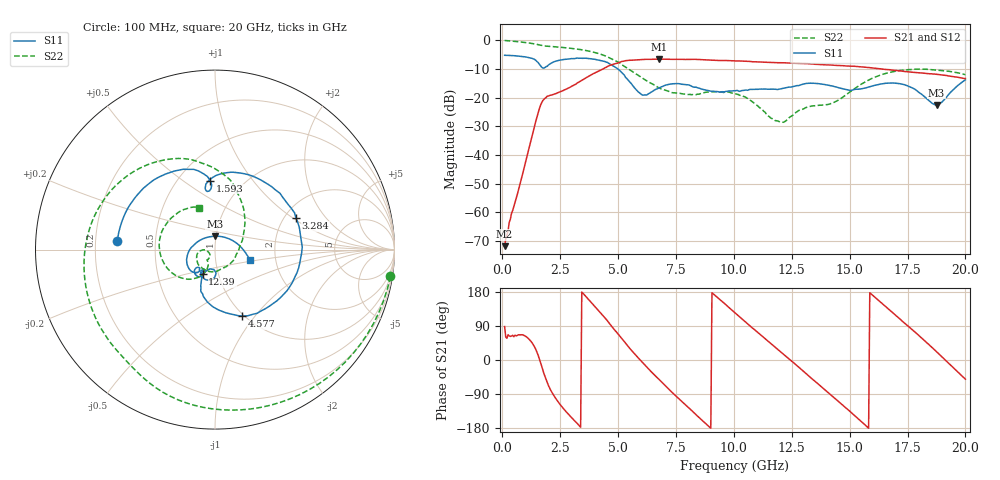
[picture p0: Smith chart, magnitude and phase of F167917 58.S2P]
!  2-Port S-parameters saved by WinCal
! VAR MeasName=S-Parameters (CALIBRATED_DATA) read from VNA (N5242A)
! VAR MeasDate=2016-11-22 9:02:51
! VAR NAME=F167917 58
! VAR FILENAME=F167917 58.S2P
! VAR DATE=2016-11-22 9:02:51
! VAR PHYS_PORTS=1,2
# Hz S DB R 50
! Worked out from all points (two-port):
!   401 points, 100 MHz to 20 GHz, reference 50 ohm
!   highest |S21| = -6.60 dB at 6.766 GHz (marker M1); lowest = -71.7 dB at 100 MHz (marker M2)
!   |S21| within 3 dB of the highest: 4.441 GHz to 15.89 GHz (11.45 GHz wide, 113 % of centre)
!   lowest |S11| = -22.5 dB at 18.76 GHz (marker M3), VSWR 1.16, Z = 49.3 + j7.4 ohm
!   |S11| at or under -10 dB: 4.985 GHz to end of sweep
!   |S22| runs from -28.6 to -0.1 dB; largest |S21 - S12| = 0.0034
!   S11 on the Smith chart (normalised r, x): 100 MHz: 0.29, +0.04; 1.593 GHz: 0.71, +0.64; 3.284 GHz: 2.30, +1.06; 4.577 GHz: 0.98, -0.86; 12.39 GHz: 0.84, -0.24; 20 GHz: 1.47, -0.18
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1e8  -5.26 174.9  -71.73 88.2  -72.43 87.3  -0.10 -8.7
8.4625e8  -5.64 136.7  -47.53 66.7  -47.58 67.3  -0.67 -66.9
1.5925e9  -8.29 93.9  -24.06 4.6  -24.07 4.6  -1.63 -115.8
2.43825e9  -7.03 74.6  -18.18 -112.7  -18.18 -112.7  -2.41 -157.3
3.284e9  -6.30 21.5  -14.70 -170.7  -14.71 -170.6  -3.16 163.6
3.43325e9  -6.31 11.4  -13.97 179.3  -13.97 179.5  -3.35 156.6
4.5775e9  -7.95 -67.7  -9.00 100.3  -8.95 100.4  -5.96 101.9
5.1745e9  -11.39 -103.8  -7.38 56.0  -7.36 56.0  -8.61 73.4
5.72175e9  -16.72 -115.1  -6.89 15.5  -6.87 15.5  -11.47 52.7
6.7665e9  -16.67 -89.7  -6.60 -51.6  -6.60 -51.6  -16.60 13.0
7.662e9  -15.19 -109.8  -6.69 -104.3  -6.68 -104.2  -18.50 -30.7
8.60725e9  -17.03 -123.1  -6.75 -157.9  -6.73 -157.9  -18.50 -81.3
1.005e10  -17.63 -116.8  -7.21 124.5  -7.21 124.6  -18.69 -149.5
1.109475e10  -17.04 -117.6  -7.57 69.6  -7.55 69.5  -23.39 -178.9
1.189075e10  -17.18 -117.1  -7.84 28.7  -7.81 28.7  -28.13 -157.0
1.238825e10  -16.32 -116.6  -8.00 2.5  -7.96 2.4  -26.99 -128.3
1.338325e10  -15.01 -125.4  -8.30 -50.0  -8.26 -49.9  -22.91 -127.6
1.43285e10  -16.11 -135.6  -8.74 -99.4  -8.70 -99.4  -21.63 -118.1
1.527375e10  -17.08 -128.6  -9.15 -149.9  -9.11 -150.2  -16.55 -115.3
1.67165e10  -14.93 -140.2  -10.28 132.4  -10.30 132.3  -11.26 -152.2
1.875625e10  -22.53 91.4  -11.90 21.5  -11.87 21.7  -10.39 146.2
2e10  -13.81 -17.2  -13.35 -50.6  -13.29 -50.3  -12.03 110.7
